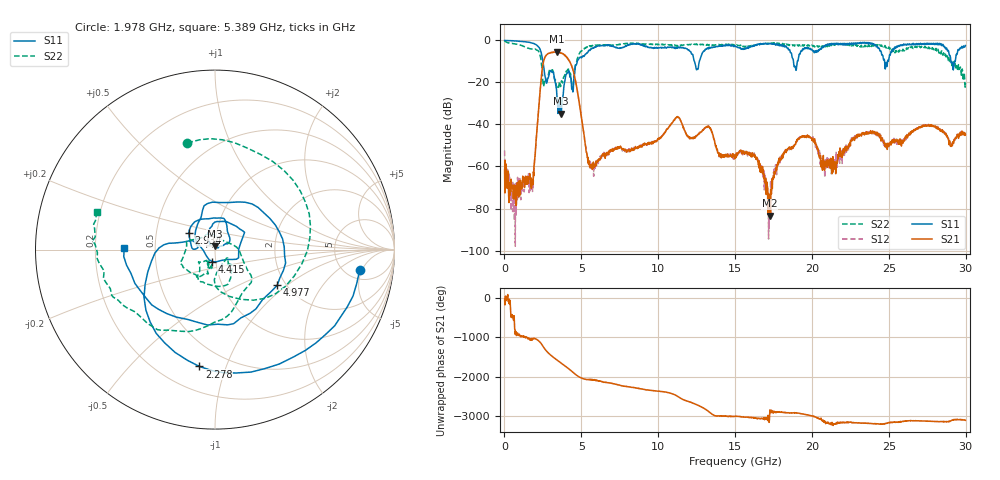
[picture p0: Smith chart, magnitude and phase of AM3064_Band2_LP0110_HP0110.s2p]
# Hz S DB R 50.0
!freq dBS11 angS11 dBS21 angS21 dBS12 angS12 dBS22 angS22
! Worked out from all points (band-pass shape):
!   1600 points, 10 MHz to 29.98 GHz, reference 50 ohm
!   highest |S21| = -5.37 dB at 3.403 GHz (marker M1); lowest = -83.4 dB at 17.25 GHz (marker M2)
!   |S21| within 3 dB of the highest: 2.615 GHz to 4.082 GHz (1.467 GHz wide, 43.8 % of centre)
!   lowest |S11| = -34.9 dB at 3.684 GHz (marker M3), VSWR 1.04, Z = 49.7 + j1.78 ohm
!   |S11| at or under -10 dB: 2.499 GHz to 4.738 GHz (2.238 GHz wide, 61.9 % of centre); 12.36 GHz to 12.67 GHz (313.9 MHz wide, 2.51 % of centre); 18.8 GHz to 19.05 GHz (249.6 MHz wide, 1.32 % of centre)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
!   |S22| runs from -23.6 to -0.2 dB; largest |S21 - S12| = 0.017
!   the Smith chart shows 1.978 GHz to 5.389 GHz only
!   S11 on the Smith chart (normalised r, x): 1.978 GHz: 6.66, -4.53; 2.278 GHz: 0.35, -0.81; 2.934 GHz: 0.73, +0.14; 4.415 GHz: 0.96, -0.13; 4.977 GHz: 1.80, -0.85; 5.389 GHz: 0.33, +0.01
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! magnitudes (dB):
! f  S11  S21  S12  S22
! 10 MHz  0.0  -61.5  -52.4  -0.2
! 609.8 MHz  -0.2  -70.8  -82.0  -1.6
! 1.978 GHz  -1.8  -56.1  -56.2  -4.2
! 2.278 GHz  -3.7  -27.6  -27.6  -6.2
! 2.934 GHz  -15.2  -6.0  -6.0  -14.0
! 3.403 GHz  -25.4  -5.4  -5.6  -22.4
! 3.684 GHz  -34.9  -6.0  -6.0  -20.5
! 4.415 GHz  -23.3  -13.1  -12.9  -21.6
! 4.977 GHz  -8.0  -35.1  -35.1  -5.2
! 5.015 GHz  -8.3  -36.9  -36.9  -5.1
! 5.389 GHz  -5.9  -55.8  -54.8  -3.2
! 10 GHz  -3.5  -46.6  -47.1  -1.9
! 11.27 GHz  -3.5  -36.4  -36.2  -2.5
! 15 GHz  -2.6  -55.2  -54.8  -2.0
! 16.3 GHz  -2.1  -54.8  -54.6  -2.2
! 17.25 GHz  -1.4  -83.4  -73.5  -1.3
! 18.19 GHz  -2.3  -53.9  -52.6  -1.9
! 19.99 GHz  -4.3  -46.8  -46.8  -2.2
! 21.43 GHz  -2.0  -59.8  -59.4  -1.8
! 23.25 GHz  -1.2  -44.0  -44.4  -3.2
! 25 GHz  -9.0  -50.4  -49.7  -3.2
! 29.98 GHz  -2.4  -45.1  -45.2  -20.3
